(* Logix 5000 AddOnInstructionDefinition export YAI_Assy_170_116_EIP_Hz; software revision 21.03 *)

ADD_ON_INSTRUCTION YAI_Assy_170_116_EIP_Hz   (* revision 1.0, vendor Yaskawa America, Inc. *)
// YAI Assembly 170 and 116
// Help:
// This add-on instruction is for use with input assembly 170 and output assembly 116.
// Node_Input_Assy is defined as the node's input assembly integer array.
// Node_Output_Assy is defined as the node's output assembly integer array.
// Torque limit/reference, torque compensation and torque output variables are only available with A1000.
VAR_IN_OUT
   Node_Input_Assy : AB:ETHERNET_MODULE_INT_24Bytes:I:0; {required}   // Input assembly words
   Node_Output_Assy : AB:ETHERNET_MODULE_INT_44Bytes:O:0; {required}   // Output assembly words
END_VAR
VAR_OUTPUT
   Running : BOOL; {access Read Only, visible}   // Drive running forward status bit
   ZSP : BOOL; {access Read Only, visible}   // Drive zero speed status bit
   RunningRev : BOOL; {access Read Only, visible}   // Drive running reverse status bit
   Reset : BOOL; {access Read Only, visible}   // Drive reset command status bit
   At_Speed : BOOL; {access Read Only, visible}   // Drive at commanded speed status bit
   Ready : BOOL; {access Read Only, visible}   // Drive ready status bit
   Alarm : BOOL; {access Read Only, visible}   // Drive alarm status bit
   Faulted : BOOL; {access Read Only, visible}   // Drive faulted status bit
   OPE : BOOL; {access Read Only}   // OPE alarm/fault present
   UV : BOOL; {access Read Only}   // Drive in UV (undervoltage) state status bit
   NetCtrlStatus : BOOL; {access Read Only, visible}   // Drive network run source status bit (1 = source coming from network)
   MFO_1_Status : BOOL; {access Read Only, visible}   // Drive multi-function output 1 (M1-M2 for A/P1000, MA/MB/MC for V1000) status
   MFO_2_Status : BOOL; {access Read Only, visible}   // Drive multi-function output 1 (M3-M4 for A/P1000, P1 for V1000) status
   MFO_3_Status : BOOL; {access Read Only, visible}   // Drive multi-function output 1 (M5-M6 for A/P1000, P2 for V1000) status
   ZSV : BOOL; {access Read Only, visible}   // Drive zero servo completed status bit
   Motor_Speed : REAL; {access Read Only, visible}   // Motor speed in Hz (xx.xx resolution)
   Custom_In_1 : INT; {access Read Only}
   Custom_In_2 : INT; {access Read Only}
   Custom_In_3 : INT; {access Read Only}
   Custom_In_4 : INT; {access Read Only}
   Custom_In_5 : INT; {access Read Only}
   Custom_In_6 : INT; {access Read Only}
   Custom_In_7 : INT; {access Read Only}
   Custom_In_8 : INT; {access Read Only}
   Custom_In_9 : INT; {access Read Only}
   Custom_In_10 : INT; {access Read Only}
END_VAR
VAR_INPUT
   Analog_Output_1 : REAL;   // Analog output 1 level command
   Analog_Output_2 : REAL;   // Analog output 2 level command
   Custom_Out_1 : INT; {visible}   // Custom output 1 - F7-23
   Custom_Out_2 : INT; {visible}   // Custom output 2 - F7-24
   Custom_Out_3 : INT; {visible}   // Custom output 3 - F7-25
   Custom_Out_4 : INT;   // Custom output 4 - F7-26
   Custom_Out_5 : INT;   // Custom output 5 - F7-27
   Custom_Out_6 : INT;   // Custom output 6 - F7-28
   Custom_Out_7 : INT;   // Custom output 7 - F7-29
   Custom_Out_8 : INT;   // Custom output 8 - F7-30
   Custom_Out_9 : INT;   // Custom output 9 - F7-31
   Custom_Out_10 : INT;   // Custom output 10 - F7-32
   Digital_Output_1 : BOOL;   // Digital output 1 activation - M1-M2
   Digital_Output_2 : BOOL;   // Digital output 2 activation - M3-M4
   Digital_Output_3 : BOOL;   // Digital output 3 activation - M5-M6
   Digital_Output_Fault : BOOL;   // Fault relay activation - MA-MB-MC
   Digital_Output_Fault_Enable : BOOL;   // Bit to enable control of fault output relay over the network
   External_Fault : BOOL;   // External fault command (EF0)
   FaultReset : BOOL; {visible}   // Fault reset command
   Freq_Ref : REAL; {visible}   // Frequency reference command in Hz (xx.xx resolution)
   MFI_3 : BOOL; {visible}   // Multi-function input 3
   MFI_4 : BOOL; {visible}   // Multi-function input 4
   MFI_5 : BOOL; {visible}   // Multi-function input 5
   MFI_6 : BOOL; {visible}   // Multi-function input 6
   MFI_7 : BOOL; {visible}   // Multi-function input 7
   MFI_8 : BOOL; {visible}   // Multi-function input 8
   MFO_1 : BOOL; {visible}   // Multi-function output (M1-M2 for A/P1000, MA/MB/MC for V1000)
   MFO_2 : BOOL; {visible}   // Multi-function output (M3-M4 for A/P1000, P1 for V1000)
   MFO_3 : BOOL; {visible}   // Multi-function output (M5-M6 for A/P1000, P2 for V1000)
   Net_Control : BOOL;   // Network start/stop control bit
   Net_Ref : BOOL;   // Network reference control bit
   RunFwd : BOOL; {visible}   // Forward run command
   RunRev : BOOL; {visible}   // Reverse run command
   Torq_Comp : REAL; {visible}   // Torque compensation command (A1000 only)
   Torq_Ref_Limit : REAL; {visible}   // Torque reference/limit (A1000 only)
END_VAR
VAR
   FRef_Convert : DINT;
   FOut_Convert : REAL;
   FOut_Temp : REAL;
   TRef_Convert : INT;
   TComp_Convert : INT;
   TOut_Convert : REAL;
   TOut_Temp : REAL;
   IOut_Temp : REAL;
   IOut_Convert : REAL;
   AO1_Convert : INT;
   AO2_Convert : INT;
   Motor_Speed_Temp : REAL;
   Motor_Speed_Convert : REAL;
   Freq_Cmd_Temp : REAL;
   Freq_Cmd_Convert : REAL;
   AI1_Temp : REAL;
   AI1_Convert : REAL;
   AI2_Temp : REAL; {access None}
   AI2_Convert : REAL; {access None}
   AI3_Temp : REAL; {access None}
   AI3_Convert : REAL; {access None}
END_VAR

ROUTINE Logic   (* ladder *)
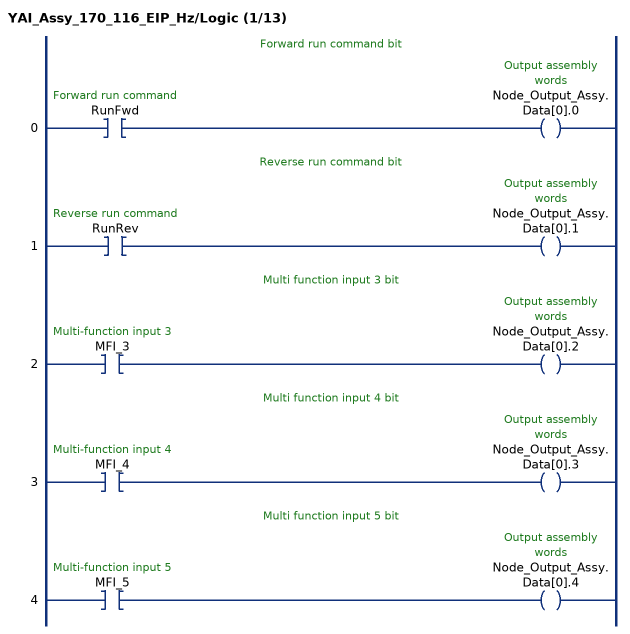
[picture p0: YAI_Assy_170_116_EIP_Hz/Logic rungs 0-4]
   // Forward run command bit
   0: XIC(RunFwd)OTE(Node_Output_Assy.Data[0].0);
   // Reverse run command bit
   1: XIC(RunRev)OTE(Node_Output_Assy.Data[0].1);
   // Multi function input 3 bit
   2: XIC(MFI_3)OTE(Node_Output_Assy.Data[0].2);
   // Multi function input 4 bit
   3: XIC(MFI_4)OTE(Node_Output_Assy.Data[0].3);
   // Multi function input 5 bit
   4: XIC(MFI_5)OTE(Node_Output_Assy.Data[0].4);
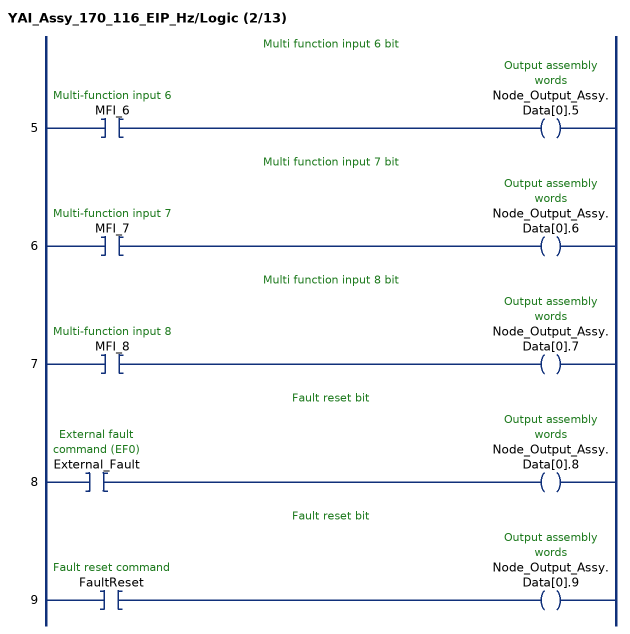
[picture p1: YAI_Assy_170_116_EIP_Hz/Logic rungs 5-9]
   // Multi function input 6 bit
   5: XIC(MFI_6)OTE(Node_Output_Assy.Data[0].5);
   // Multi function input 7 bit
   6: XIC(MFI_7)OTE(Node_Output_Assy.Data[0].6);
   // Multi function input 8 bit
   7: XIC(MFI_8)OTE(Node_Output_Assy.Data[0].7);
   // Fault reset bit
   8: XIC(External_Fault)OTE(Node_Output_Assy.Data[0].8);
   // Fault reset bit
   9: XIC(FaultReset)OTE(Node_Output_Assy.Data[0].9);
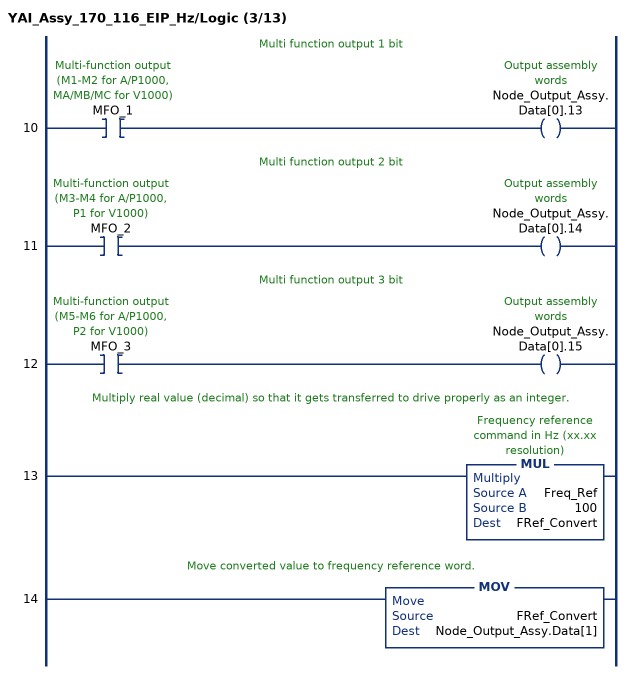
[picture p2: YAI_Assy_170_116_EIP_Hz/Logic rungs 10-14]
   // Multi function output 1 bit
   10: XIC(MFO_1)OTE(Node_Output_Assy.Data[0].13);
   // Multi function output 2 bit
   11: XIC(MFO_2)OTE(Node_Output_Assy.Data[0].14);
   // Multi function output 3 bit
   12: XIC(MFO_3)OTE(Node_Output_Assy.Data[0].15);
   // Multiply real value (decimal) so that it gets transferred to drive properly as an integer.
   13: MUL(Freq_Ref,100,FRef_Convert);
   // Move converted value to frequency reference word.
   14: MOV(FRef_Convert,Node_Output_Assy.Data[1]);
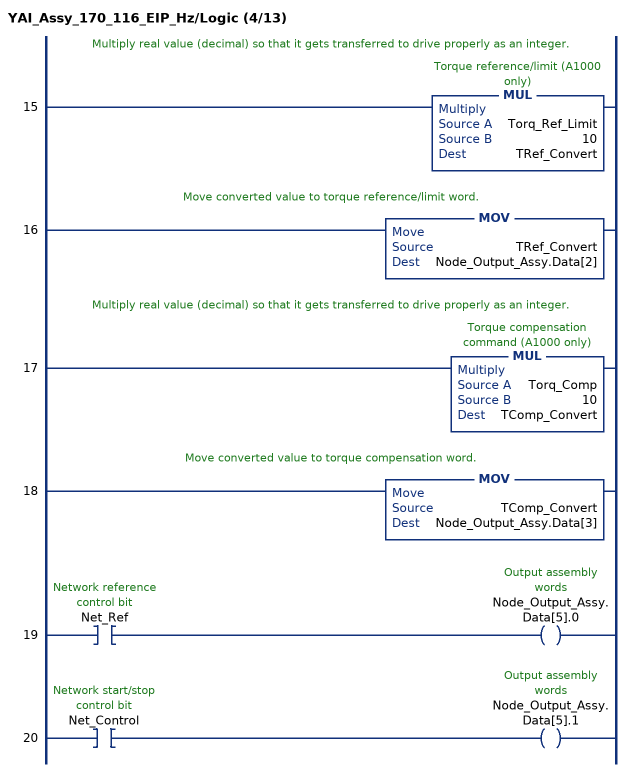
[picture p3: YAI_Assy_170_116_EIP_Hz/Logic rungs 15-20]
   // Multiply real value (decimal) so that it gets transferred to drive properly as an integer.
   15: MUL(Torq_Ref_Limit,10,TRef_Convert);
   // Move converted value to torque reference/limit word.
   16: MOV(TRef_Convert,Node_Output_Assy.Data[2]);
   // Multiply real value (decimal) so that it gets transferred to drive properly as an integer.
   17: MUL(Torq_Comp,10,TComp_Convert);
   // Move converted value to torque compensation word.
   18: MOV(TComp_Convert,Node_Output_Assy.Data[3]);
   19: XIC(Net_Ref)OTE(Node_Output_Assy.Data[5].0);
   20: XIC(Net_Control)OTE(Node_Output_Assy.Data[5].1);
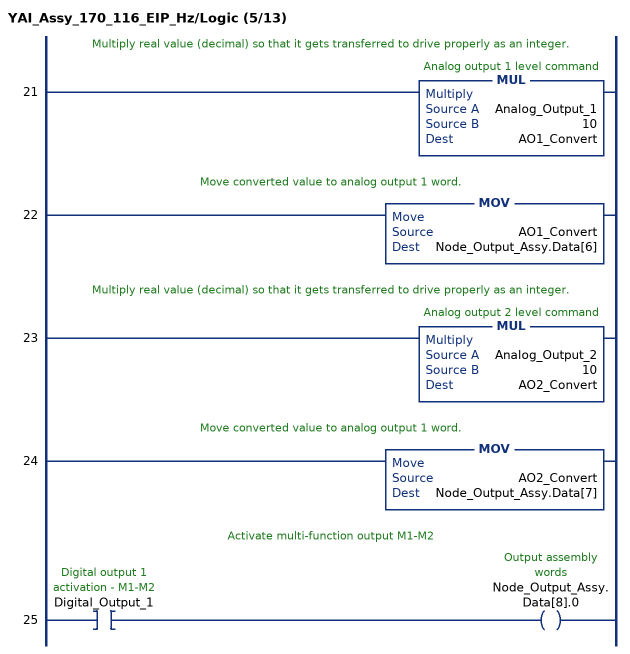
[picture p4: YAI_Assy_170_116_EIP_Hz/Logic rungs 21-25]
   // Multiply real value (decimal) so that it gets transferred to drive properly as an integer.
   21: MUL(Analog_Output_1,10,AO1_Convert);
   // Move converted value to analog output 1 word.
   22: MOV(AO1_Convert,Node_Output_Assy.Data[6]);
   // Multiply real value (decimal) so that it gets transferred to drive properly as an integer.
   23: MUL(Analog_Output_2,10,AO2_Convert);
   // Move converted value to analog output 1 word.
   24: MOV(AO2_Convert,Node_Output_Assy.Data[7]);
   // Activate multi-function output M1-M2
   25: XIC(Digital_Output_1)OTE(Node_Output_Assy.Data[8].0);
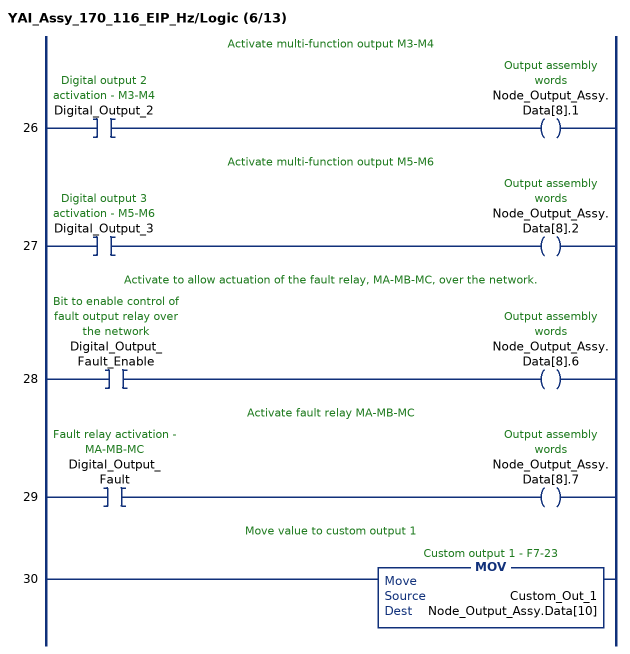
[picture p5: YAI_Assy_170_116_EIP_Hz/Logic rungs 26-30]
   // Activate multi-function output M3-M4
   26: XIC(Digital_Output_2)OTE(Node_Output_Assy.Data[8].1);
   // Activate multi-function output M5-M6
   27: XIC(Digital_Output_3)OTE(Node_Output_Assy.Data[8].2);
   // Activate to allow actuation of the fault relay, MA-MB-MC, over the network.
   28: XIC(Digital_Output_Fault_Enable)OTE(Node_Output_Assy.Data[8].6);
   // Activate fault relay MA-MB-MC
   29: XIC(Digital_Output_Fault)OTE(Node_Output_Assy.Data[8].7);
   // Move value to custom output 1
   30: MOV(Custom_Out_1,Node_Output_Assy.Data[10]);
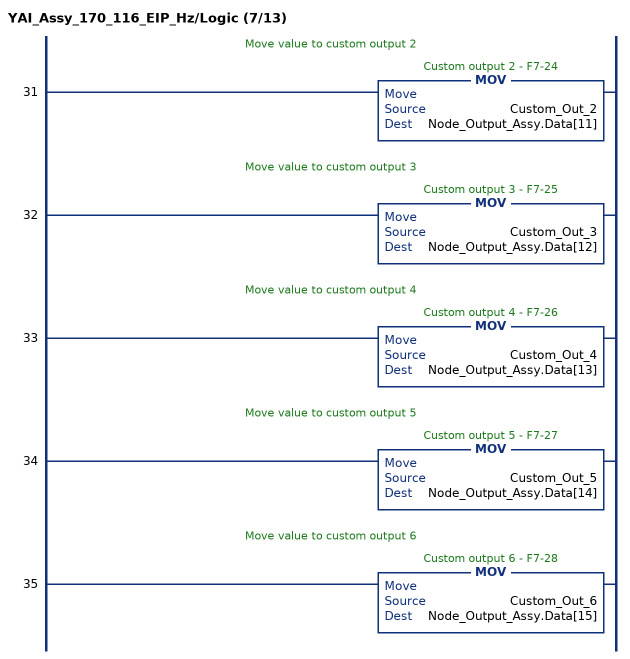
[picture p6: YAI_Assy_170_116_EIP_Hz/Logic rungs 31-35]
   // Move value to custom output 2
   31: MOV(Custom_Out_2,Node_Output_Assy.Data[11]);
   // Move value to custom output 3
   32: MOV(Custom_Out_3,Node_Output_Assy.Data[12]);
   // Move value to custom output 4
   33: MOV(Custom_Out_4,Node_Output_Assy.Data[13]);
   // Move value to custom output 5
   34: MOV(Custom_Out_5,Node_Output_Assy.Data[14]);
   // Move value to custom output 6
   35: MOV(Custom_Out_6,Node_Output_Assy.Data[15]);
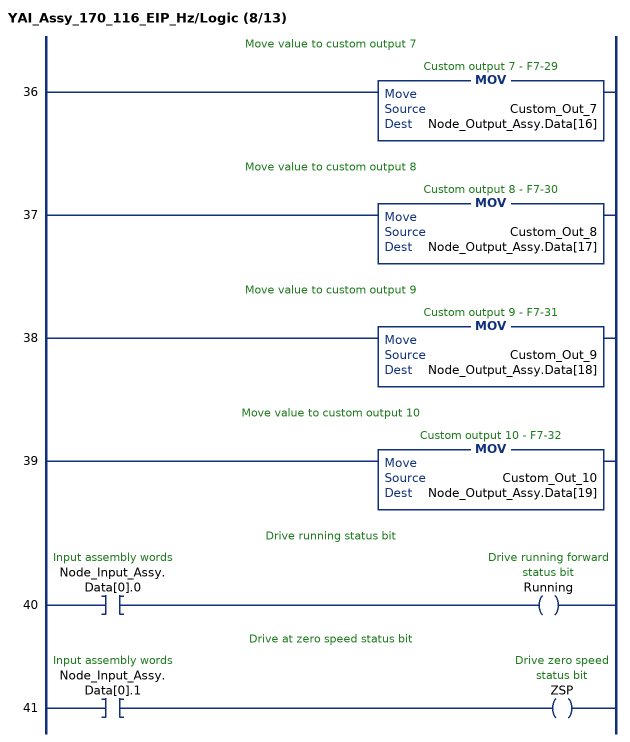
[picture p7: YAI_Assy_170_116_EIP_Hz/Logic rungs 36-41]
   // Move value to custom output 7
   36: MOV(Custom_Out_7,Node_Output_Assy.Data[16]);
   // Move value to custom output 8
   37: MOV(Custom_Out_8,Node_Output_Assy.Data[17]);
   // Move value to custom output 9
   38: MOV(Custom_Out_9,Node_Output_Assy.Data[18]);
   // Move value to custom output 10
   39: MOV(Custom_Out_10,Node_Output_Assy.Data[19]);
   // Drive running status bit
   40: XIC(Node_Input_Assy.Data[0].0)OTE(Running);
   // Drive at zero speed status bit
   41: XIC(Node_Input_Assy.Data[0].1)OTE(ZSP);
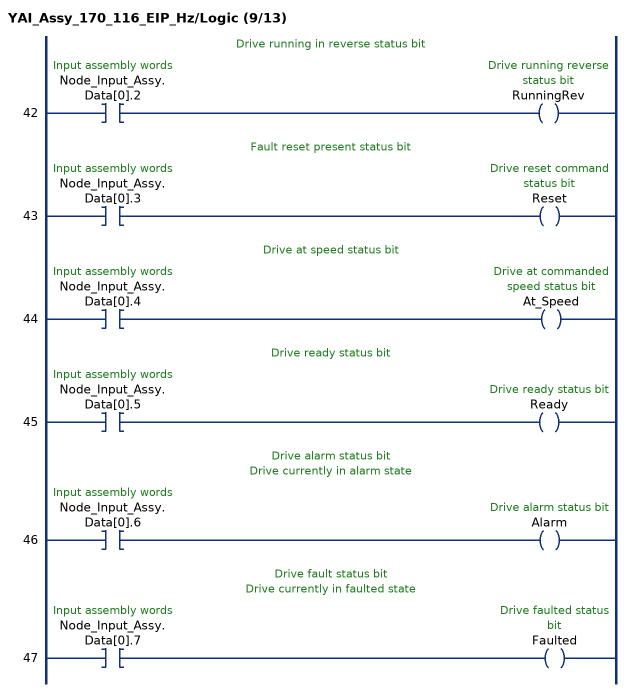
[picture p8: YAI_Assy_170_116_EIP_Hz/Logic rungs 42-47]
   // Drive running in reverse status bit
   42: XIC(Node_Input_Assy.Data[0].2)OTE(RunningRev);
   // Fault reset present status bit
   43: XIC(Node_Input_Assy.Data[0].3)OTE(Reset);
   // Drive at speed status bit
   44: XIC(Node_Input_Assy.Data[0].4)OTE(At_Speed);
   // Drive ready status bit
   45: XIC(Node_Input_Assy.Data[0].5)OTE(Ready);
   // Drive alarm status bit
   // Drive currently in alarm state
   46: XIC(Node_Input_Assy.Data[0].6)OTE(Alarm);
   // Drive fault status bit
   // Drive currently in faulted state
   47: XIC(Node_Input_Assy.Data[0].7)OTE(Faulted);
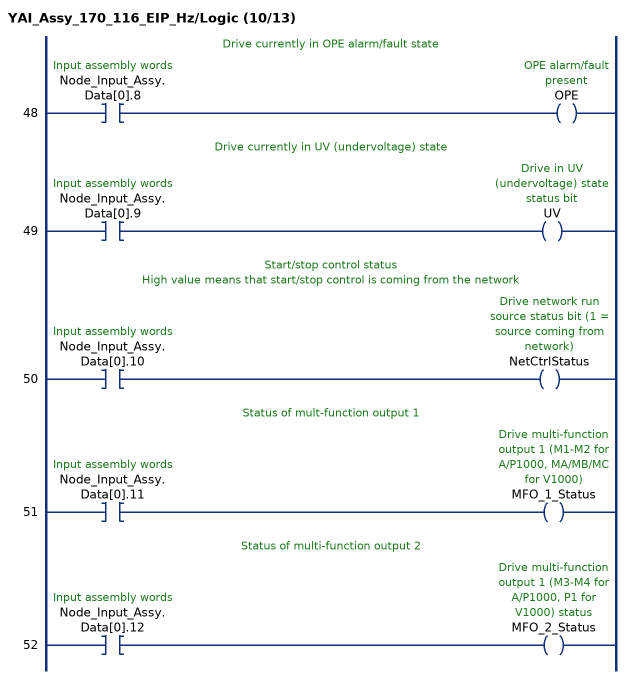
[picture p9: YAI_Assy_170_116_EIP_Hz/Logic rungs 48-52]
   // Drive currently in OPE alarm/fault state
   48: XIC(Node_Input_Assy.Data[0].8)OTE(OPE);
   // Drive currently in UV (undervoltage) state
   49: XIC(Node_Input_Assy.Data[0].9)OTE(UV);
   // Start/stop control status
   // High value means that start/stop control is coming from the network
   50: XIC(Node_Input_Assy.Data[0].10)OTE(NetCtrlStatus);
   // Status of mult-function output 1
   51: XIC(Node_Input_Assy.Data[0].11)OTE(MFO_1_Status);
   // Status of multi-function output 2
   52: XIC(Node_Input_Assy.Data[0].12)OTE(MFO_2_Status);
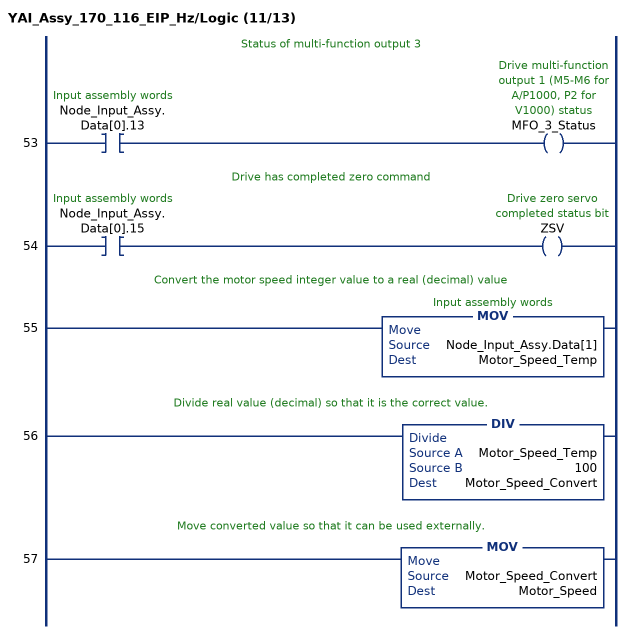
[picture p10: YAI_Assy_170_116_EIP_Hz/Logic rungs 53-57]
   // Status of multi-function output 3
   53: XIC(Node_Input_Assy.Data[0].13)OTE(MFO_3_Status);
   // Drive has completed zero command
   54: XIC(Node_Input_Assy.Data[0].15)OTE(ZSV);
   // Convert the motor speed integer value to a real (decimal) value
   55: MOV(Node_Input_Assy.Data[1],Motor_Speed_Temp);
   // Divide real value (decimal) so that it is the correct value.
   56: DIV(Motor_Speed_Temp,100,Motor_Speed_Convert);
   // Move converted value so that it can be used externally.
   57: MOV(Motor_Speed_Convert,Motor_Speed);
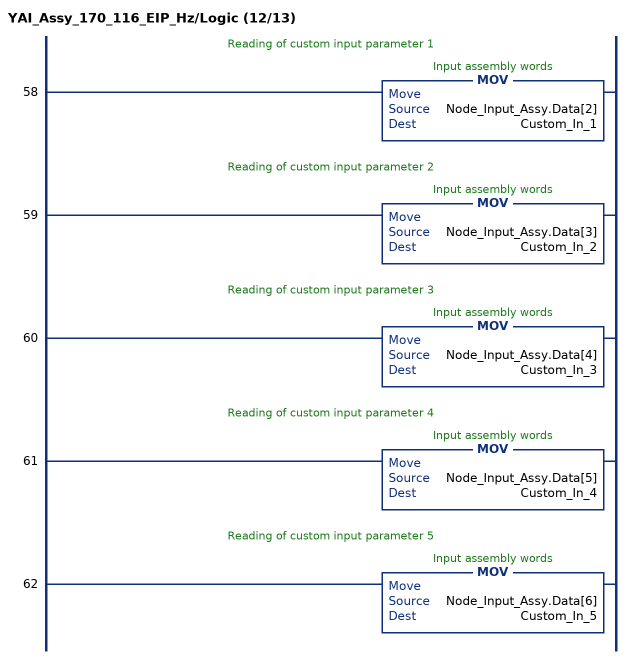
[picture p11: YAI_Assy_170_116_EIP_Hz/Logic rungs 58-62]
   // Reading of custom input parameter 1
   58: MOV(Node_Input_Assy.Data[2],Custom_In_1);
   // Reading of custom input parameter 2
   59: MOV(Node_Input_Assy.Data[3],Custom_In_2);
   // Reading of custom input parameter 3
   60: MOV(Node_Input_Assy.Data[4],Custom_In_3);
   // Reading of custom input parameter 4
   61: MOV(Node_Input_Assy.Data[5],Custom_In_4);
   // Reading of custom input parameter 5
   62: MOV(Node_Input_Assy.Data[6],Custom_In_5);
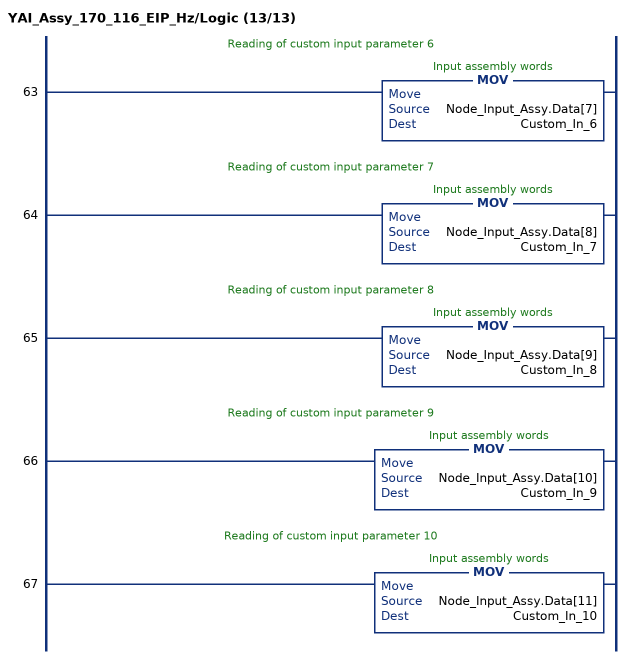
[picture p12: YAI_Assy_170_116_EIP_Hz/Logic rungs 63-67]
   // Reading of custom input parameter 6
   63: MOV(Node_Input_Assy.Data[7],Custom_In_6);
   // Reading of custom input parameter 7
   64: MOV(Node_Input_Assy.Data[8],Custom_In_7);
   // Reading of custom input parameter 8
   65: MOV(Node_Input_Assy.Data[9],Custom_In_8);
   // Reading of custom input parameter 9
   66: MOV(Node_Input_Assy.Data[10],Custom_In_9);
   // Reading of custom input parameter 10
   67: MOV(Node_Input_Assy.Data[11],Custom_In_10);
END_ROUTINE
END_ADD_ON_INSTRUCTION
